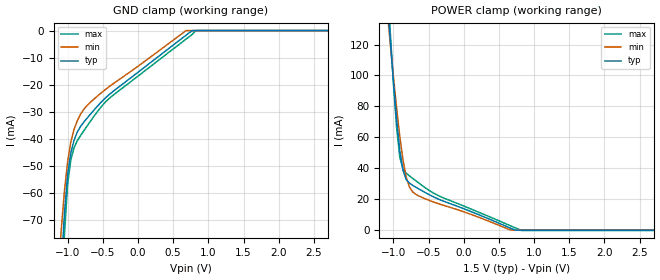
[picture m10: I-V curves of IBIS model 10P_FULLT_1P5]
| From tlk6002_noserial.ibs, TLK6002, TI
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[Model]   10P_FULLT_1P5
Model_type   Input
Polarity   Non-Inverting
Vinh =  0.85
Vinl =  0.65
C_comp   2.108887p   1.924381p   2.428843p
[Model Spec]
Vinh   0.85   0.775   0.925
Vinl   0.65   0.575   0.725
[Temperature Range]   25   125   -40
[Voltage Range]   1.5   1.35   1.65
[POWER_clamp]
-1.5V     438.6mA    364.7mA    521.4mA
-1.091V   152.5mA    143.5mA    164.4mA
-1.045V   123.5mA    120.9mA    128.4mA
-954.5mV  71.46mA    78.92mA    66.31mA
-909.1mV  51.36mA    60.6mA     47.11mA
-863.6mV  38.48mA    45.3mA     39.43mA
-818.2mV  32.78mA    34.25mA    36.82mA
-772.7mV  30.47mA    27.86mA    35.09mA
-681.8mV  27.79mA    23.15mA    31.9mA
-363.6mV  20.14mA    17.16mA    22.36mA
818.2mV   0A         0A         -211.9uA
3V        0A         0A         -211.9uA
[GND_clamp]
-1.5V     -363.8mA   -265.2mA   -482mA
-1.091V   -88.46mA   -73.81mA   -104.5mA
-1.045V   -67.78mA   -59.43mA   -75.49mA
-1V       -53.37mA   -48.5mA    -56.76mA
-954.5mV  -45.18mA   -41.17mA   -47.82mA
-909.1mV  -40.56mA   -36.52mA   -43.33mA
-863.6mV  -37.54mA   -33.36mA   -40.72mA
-772.7mV  -33.89mA   -29.18mA   -37.11mA
-409.1mV  -23.62mA   -20.69mA   -25.05mA
681.8mV   -1.746mA   0A         -3.188mA
818.2mV   0A         0A         0A
3V        0A         0A         0A
